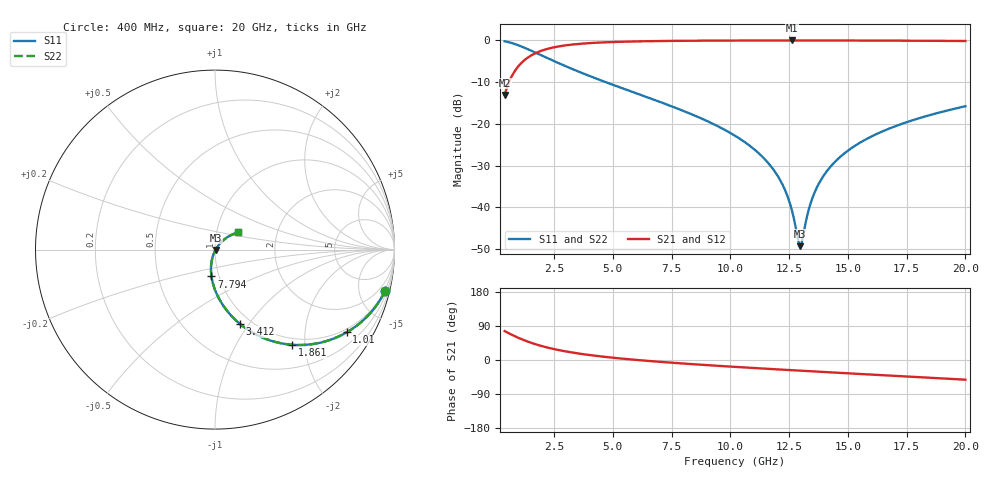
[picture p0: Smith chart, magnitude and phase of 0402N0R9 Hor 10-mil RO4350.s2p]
# GHz S MA R 50
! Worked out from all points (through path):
!   1960 points, 400 MHz to 20 GHz, reference 50 ohm
!   highest |S21| = -0.03 dB at 12.63 GHz (marker M1); lowest = -13.1 dB at 400 MHz (marker M2)
!   lowest |S11| = -49.3 dB at 12.98 GHz (marker M3), VSWR 1.01, Z = 50.3 - j0.155 ohm
!   |S11| at or under -10 dB: 4.689 GHz to end of sweep
!   |S22| runs from -49.3 to -0.2 dB; largest |S21 - S12| = 0
!   S11 on the Smith chart (normalised r, x): 400 MHz: 0.88, -8.26; 1.01 GHz: 0.88, -3.26; 1.861 GHz: 0.88, -1.74; 3.412 GHz: 0.89, -0.91; 7.794 GHz: 0.92, -0.28; 20 GHz: 1.27, +0.25
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0.4  0.9752 -13.7  0.221 76.3  0.221 76.3  0.9752 -13.7
1.010311  0.8667 -32.1  0.4983 57.9  0.4983 57.9  0.8667 -32.1
1.860745  0.6816 -51.1  0.7307 38.9  0.7307 38.9  0.6816 -51.1
2.571108  0.5525 -62.0  0.8321 27.9  0.8321 27.9  0.5525 -62.0
3.411536  0.4372 -71.4  0.8977 18.4  0.8977 18.4  0.4372 -71.4
3.671669  0.4082 -73.8  0.9111 16.0  0.9111 16.0  0.4082 -73.8
6.943338  0.1856 -93.8  0.9799 -4.5  0.9799 -4.5  0.1856 -93.8
7.793772  0.1506 -97.5  0.9857 -8.4  0.9857 -8.4  0.1506 -97.5
10.205  0.0718 -105.8  0.994 -18.2  0.994 -18.2  0.0718 -105.8
11.10546  0.04709 -107.7  0.9953 -21.5  0.9953 -21.5  0.04709 -107.7
11.78581  0.0295 -107.7  0.9958 -24.0  0.9958 -24.0  0.0295 -107.7
12.27606  0.01733 -104.7  0.996 -25.7  0.996 -25.7  0.01733 -104.7
12.62624  0.009047 -95.2  0.9961 -27.0  0.9961 -27.0  0.009047 -95.2
12.88637  0.00399 -59.4  0.9961 -27.9  0.9961 -27.9  0.00399 -59.4
12.97642  0.003416 -26.8  0.996 -28.2  0.996 -28.2  0.003416 -26.8
13.05646  0.003972 1.9  0.996 -28.5  0.996 -28.5  0.003972 1.9
13.46667  0.01229 43.6  0.9959 -29.9  0.9959 -29.9  0.01229 43.6
13.9269  0.02288 49.6  0.9956 -31.5  0.9956 -31.5  0.02288 49.6
14.59724  0.03834 50.7  0.995 -33.8  0.995 -33.8  0.03834 50.7
15.51771  0.05938 49.4  0.9938 -36.9  0.9938 -36.9  0.05938 49.4
16.73834  0.08711 46.4  0.9915 -41.0  0.9915 -41.0  0.08711 46.4
20  0.1622 36.5  0.9814 -51.9  0.9814 -51.9  0.1622 36.5
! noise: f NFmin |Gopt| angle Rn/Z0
0.4  0.001398  0.8383  5.74  0.001826
2.571  0.005107  0.6847  8.481  0.003125
4.752  0.008095  0.6394  12.39  0.00419
6.933  0.01078  0.612  16.57  0.005054
9.104  0.01328  0.5931  20.77  0.005805
11.29  0.01569  0.5797  24.97  0.006494
13.47  0.01804  0.5701  29.1  0.007143
15.64  0.02035  0.5638  33.13  0.007768
17.82  0.02266  0.56  37.08  0.008389
20  0.02499  0.5585  40.93  0.009015
